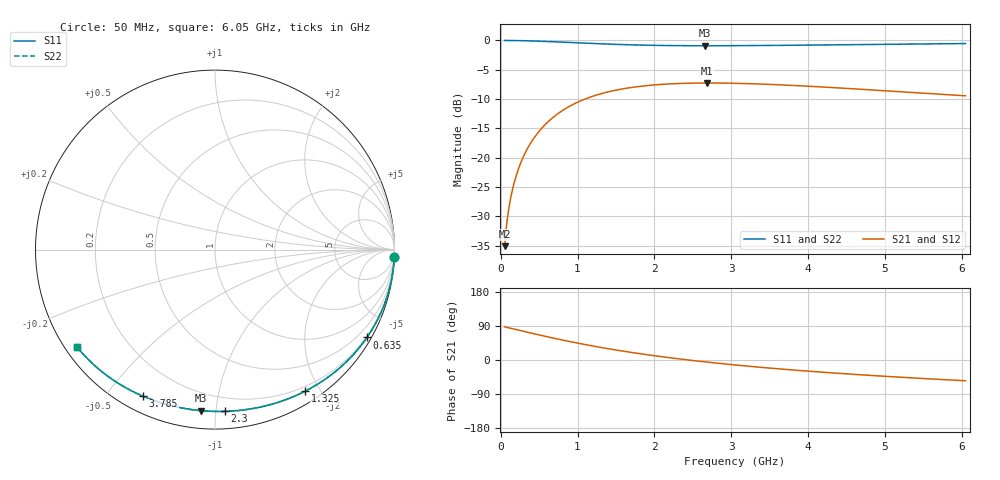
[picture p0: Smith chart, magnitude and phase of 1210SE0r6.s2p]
! AVX Thin Film Operation		Date: August 2001
! Description: Accu-P® Series, Thin Film, SMD, RF Capacitor
! Part Number: 12101J0R6ABT
! 50 MHz  -  6.05 GHz
! Serial Measurements
# mhz S db R 50
!	S11		S21		S12		S22
!	dB	Phase	dB	Phase	dB	Phase	dB	Phase
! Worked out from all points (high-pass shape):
!   401 points, 50 MHz to 6.05 GHz, reference 50 ohm
!   highest |S21| = -7.25 dB at 2.69 GHz (marker M1); lowest = -35.1 dB at 50 MHz (marker M2)
!   |S21| within 3 dB of the highest: 1.048 GHz to end of sweep
!   lowest |S11| = -0.9 dB at 2.66 GHz (marker M3), VSWR 19.15, Z = 4.8 - j45.6 ohm
!   |S11| at or under -10 dB: nowhere
!   |S22| runs from -0.9 to 0.0 dB; largest |S21 - S12| = 0
!   S11 on the Smith chart (normalised r, x): 50 MHz: 0, -47; 635 MHz: 0.16, -3.72; 1.325 GHz: 0.14, -1.81; 2.3 GHz: 0.11, -1.06; 3.785 GHz: 0.07, -0.62; 6.05 GHz: 0.03, -0.32
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50  -0.00 -2.4  -35.07 87.6  -35.07 87.6  -0.00 -2.4
65  -0.00 -3.2  -32.79 86.8  -32.79 86.8  -0.00 -3.2
110  -0.01 -5.4  -28.24 84.7  -28.24 84.7  -0.01 -5.4
140  -0.01 -6.8  -26.15 83.2  -26.15 83.2  -0.01 -6.8
185  -0.02 -9.0  -23.76 81.0  -23.76 81.0  -0.02 -9.0
245  -0.03 -11.9  -21.36 78.1  -21.36 78.1  -0.03 -11.9
320  -0.05 -15.5  -19.11 74.5  -19.11 74.5  -0.05 -15.5
410  -0.09 -19.7  -17.07 70.3  -17.07 70.3  -0.09 -19.7
635  -0.19 -30.0  -13.63 60.0  -13.63 60.0  -0.19 -30.0
830  -0.30 -38.5  -11.72 51.5  -11.72 51.5  -0.30 -38.5
1055  -0.43 -47.6  -10.21 42.4  -10.21 42.4  -0.43 -47.6
1325  -0.58 -57.6  -9.01 32.4  -9.01 32.4  -0.58 -57.6
1670  -0.74 -69.1  -8.07 20.9  -8.07 20.9  -0.74 -69.1
2060  -0.85 -80.3  -7.52 9.6  -7.52 9.6  -0.85 -80.4
2300  -0.89 -86.6  -7.35 3.4  -7.35 3.4  -0.89 -86.6
2660  -0.91 -95.0  -7.25 -5.0  -7.25 -5.0  -0.91 -95.0
2690  -0.91 -95.6  -7.25 -5.7  -7.25 -5.7  -0.91 -95.6
3050  -0.90 -103.0  -7.30 -13.1  -7.30 -13.1  -0.90 -103.1
3785  -0.82 -116.0  -7.66 -26.1  -7.66 -26.1  -0.82 -116.1
4055  -0.78 -120.2  -7.84 -30.3  -7.84 -30.3  -0.78 -120.2
5060  -0.65 -133.7  -8.62 -43.8  -8.62 -43.8  -0.65 -133.7
6050  -0.53 -144.7  -9.43 -54.8  -9.43 -54.8  -0.53 -144.7
